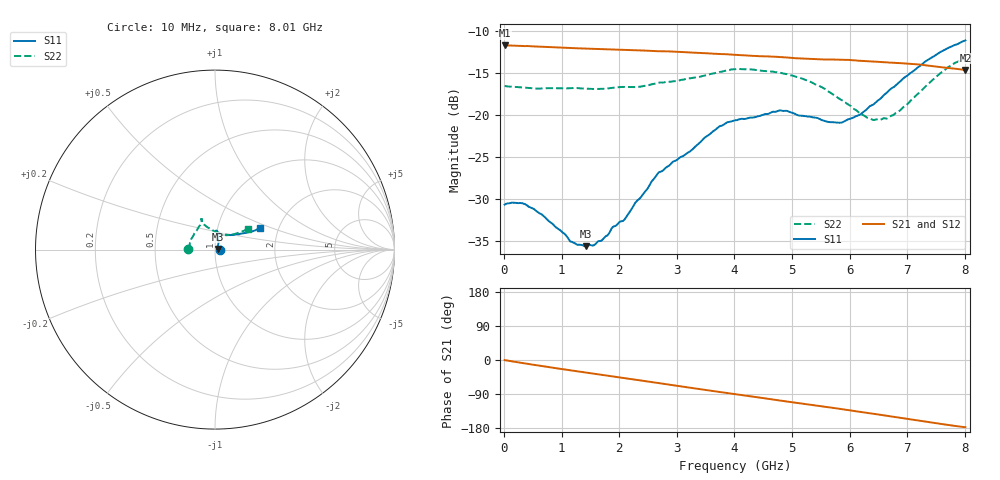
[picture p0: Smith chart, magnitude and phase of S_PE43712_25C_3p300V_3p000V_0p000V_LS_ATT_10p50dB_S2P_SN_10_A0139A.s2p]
! DEVICE ID: PE43712
! File Path: z:\PE43713\PE43713_CHAR_NOM_04292014\AMB\3p300\LS_ATT_10p50dB\PE43713_AMB_3p300V_3p000V_0p000V_LS_ATT_10p50dB_S2P_SN_10_A0139A.s2p
! Serial: 10
! Lot: A0139A
! Temp: 25C
! VDD: 3.300
! VSS: 0.000
! Control_Hi: 3.000
! Control_Lo: 0.000
! Attenuation Step: 10.50dB
! Port 1: RF1
! Port 2: RF2
! ThroughPath:1-2
! IDD: 0.0001466372
! ISS: -1.221e-007
#  Hz  S  RI  R  50
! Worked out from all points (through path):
!   801 points, 10 MHz to 8.01 GHz, reference 50 ohm
!   highest |S21| = -11.67 dB at 10 MHz (marker M1); lowest = -14.6 dB at 8.01 GHz (marker M2)
!   group delay of S21, straight-line fit = 61 ps
!   lowest |S11| = -35.7 dB at 1.42 GHz (marker M3), VSWR 1.03, Z = 51.6 + j0.415 ohm
!   |S11| at or under -10 dB: start of sweep to end of sweep
!   |S22| runs from -20.6 to -13.3 dB; largest |S21 - S12| = 0.00094
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1e7  0.0292 0.000144  0.2608 -0.00145  0.2609 -0.00133  -0.1492 0.000984
3.7e8  0.0291 -0.00333  0.2551 -0.0408  0.256 -0.0411  -0.145 0.0175
6.8e8  0.0247 -0.00368  0.2452 -0.0727  0.2452 -0.0727  -0.1404 0.0325
1.17e9  0.0175 0.000776  0.2226 -0.1163  0.2227 -0.1164  -0.1343 0.0541
1.35e9  0.0164 0.00296  0.2131 -0.1308  0.2131 -0.1309  -0.1306 0.061
1.42e9  0.016 0.00402  0.2091 -0.1362  0.209 -0.1363  -0.1285 0.0644
1.7e9  0.0148 0.00994  0.1918 -0.1567  0.1918 -0.1567  -0.1209 0.0771
1.89e9  0.0152 0.0151  0.179 -0.1695  0.179 -0.1695  -0.1165 0.0872
2.09e9  0.0145 0.0188  0.1646 -0.1819  0.1646 -0.1818  -0.1125 0.0948
2.68e9  0.02 0.0406  0.1173 -0.2102  0.1173 -0.2102  -0.0902 0.1274
3.72e9  0.0148 0.0831  0.0251 -0.2305  0.0249 -0.2305  -0.075 0.1636
4.01e9  0.0119 0.0922  -0.000562 -0.2293  -0.000584 -0.2292  -0.0777 0.1712
4.79e9  0.00726 0.1063  -0.0644 -0.2125  -0.0644 -0.2127  -0.0738 0.1633
5.35e9  0.0174 0.0955  -0.1038 -0.1899  -0.1038 -0.1898  -0.0642 0.1426
5.88e9  0.0394 0.0816  -0.1378 -0.1638  -0.1375 -0.1638  -0.0303 0.1182
6.18e9  0.0607 0.0802  -0.1539 -0.1443  -0.1536 -0.1443  -0.00322 0.1018
6.39e9  0.0803 0.0816  -0.1632 -0.1303  -0.1629 -0.1302  0.0176 0.0923
6.68e9  0.1123 0.0833  -0.1746 -0.1093  -0.1743 -0.1093  0.0499 0.083
6.99e9  0.146 0.089  -0.1842 -0.0856  -0.1839 -0.0856  0.0809 0.082
7.36e9  0.19 0.0983  -0.1895 -0.0555  -0.1893 -0.0555  0.1224 0.0913
7.72e9  0.2277 0.109  -0.189 -0.0279  -0.1889 -0.028  0.1624 0.1065
8.01e9  0.2516 0.1207  -0.1857 -0.00825  -0.1854 -0.00856  0.183 0.1169
